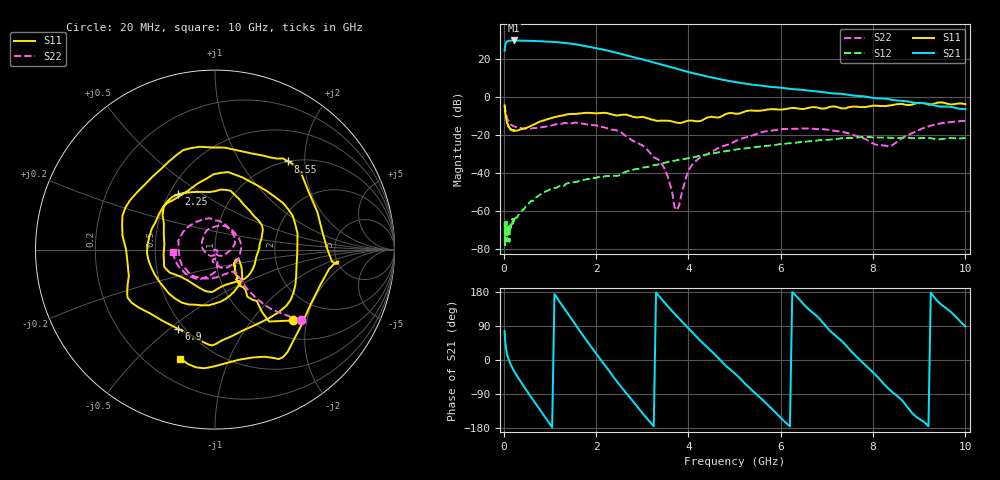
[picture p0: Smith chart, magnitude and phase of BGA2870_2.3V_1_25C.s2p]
#  HZ  S  RI  R  50.0000
! Rohde & Schwarz ZVA/B
! Temperature 25C
! Device number 1
! Measured Vcc 2.300000
! Measured Icc 0.013200
! DeltaGain  -0.201967  3dBBWHighMHz 1925.88  3dBBWLowMHz 26.83
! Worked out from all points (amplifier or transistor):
!   242 points, 20 MHz to 10 GHz, reference 50 ohm
!   highest |S21| = 29.5 dB at 230 MHz (marker M1)
!   |S21| within 3 dB of that: 30.56 MHz to 1.786 GHz (1.755 GHz wide, 193 % of centre)
!   unconditionally stable (mu >= 1): start of sweep to end of sweep
!   at 220 MHz: K = 25.83, MAG = 29.6 dB, |S12| = -64.1 dB
!   at 4 GHz: K = 4.45, MAG = 13.2 dB, |S12| = -32.3 dB
!   at 10 GHz: K = 7.24, MAG = -4.0 dB, |S12| = -21.6 dB
!   S11 on the Smith chart (normalised r, x): 20 MHz: 1.38, -1.66; 2.25 GHz: 0.56, +0.40; 6.9 GHz: 0.46, -0.54; 8.55 GHz: 1.00, +1.66; 10 GHz: 0.33, -0.68
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2e7  0.4334 -0.3948  3.903 15.59  0.000374 0.000122  0.4782 -0.3942
4.5e7  0.1798 -0.2621  20.6 14.64  0.000356 -0.0003  0.2552 -0.2907
7.5e7  0.1172 -0.1659  27.2 7.13  0.000152 -6.02e-05  0.1737 -0.2122
2.3e8  0.1157 -0.0643  25.7 -14.91  0.000263 0.000512  0.1104 -0.1259
4e8  0.1307 -0.0557  13.36 -26.24  0.000548 0.000894  0.079 -0.1279
6e8  0.1469 -0.0953  -4.479 -28.61  0.00126 0.00141  0.0428 -0.1413
8e8  0.1483 -0.1717  -19.59 -20.44  0.00236 0.00147  -0.001 -0.1563
1e9  0.0849 -0.2553  -27.06 -5.364  0.00366 0.000774  -0.0681 -0.1599
1.35e9  -0.1476 -0.3055  -15.99 19.65  0.00491 -0.00176  -0.1951 -0.0575
1.7e9  -0.356 -0.098  8.304 20.31  0.00391 -0.00527  -0.1585 0.1167
2e9  -0.3321 0.1521  17.98 5.476  0.00135 -0.0073  -0.0345 0.1757
2.25e9  -0.2042 0.3088  14.77 -6.368  -0.00181 -0.00817  0.0624 0.1347
2.65e9  0.0867 0.3277  0.7748 -12.13  -0.00672 -0.00857  0.0921 0.00451
3e9  0.2613 0.1363  -7.232 -6.214  -0.0132 -0.00417  0.0418 -0.0333
3.35e9  0.227 -0.0524  -7.269 1.183  -0.0164 0.00389  0.00155 -0.0224
4.2e9  -0.1192 -0.1931  2.039 3.305  0.00494 0.0271  0.00951 -0.0205
5.05e9  -0.1933 0.3005  1.818 -1.547  0.0406 -0.00963  -0.0709 0.00908
6.7e9  -0.0159 -0.5338  -0.7901 1.158  -0.0657 0.0216  0.144 0.000888
6.9e9  -0.2036 -0.4421  -0.247 1.307  -0.0565 0.0474  0.1337 -0.0455
8.35e9  0.2683 0.5239  0.1824 -0.8395  0.0751 -0.0383  0.00513 -0.0506
8.55e9  0.4083 0.4913  -0.1043 -0.779  0.0599 -0.0569  0.0134 -0.0693
1e10  -0.1953 -0.607  0.0144 0.4744  -0.0806 0.0222  -0.2321 -0.0158
